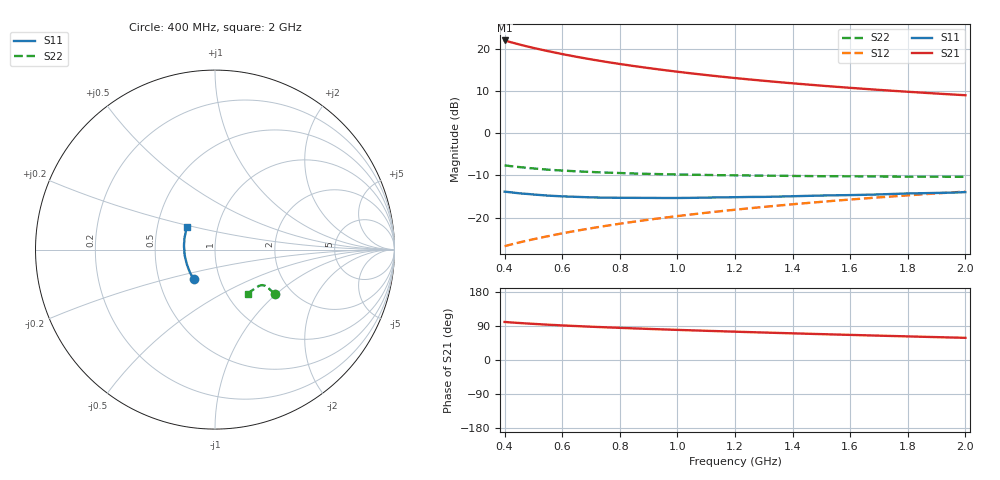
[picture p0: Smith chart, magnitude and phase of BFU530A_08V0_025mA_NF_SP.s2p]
! Filename:  P:\Prog\Test\Noise\ATS_data\Testdata_Net\06 Compressed Noise after Statistics\BFU530A_APG2013_33_A05_08p0V_025mA_NF_CM01_D.sf
! Date/Time: Tue 16/Apr/2013 15:10:58
! BFU530A_APG2013_33_A05_08p0V_1to25mA_NF_CM01_Bias8_R.sf
! Noise Parameter Data File
! BFU530A_APG2013_33_A05_08p0V_1to25mA_NF_CM01
! Date/time: Fri Apr 12 16:45:05 2013
! VAR V_out= 8.001000
! VAR I_out= 25.000000
! VAR V_in= 0.812800
! VAR I_in= 0.260050
! Device data file deembeded for feedlines and parallel
! Original file: \06 Compressed Noise after Statistics\BFU530A_APG2013_33_A05_08p0V_025mA_NF_CM01_R.sf
! Feed-files: PR017V01_150413_Feed1.s2p, PR017V01_150413_Feed2.s2p
! Parallel-file: PR017V01_150413_Par.s2p
# MHz S MA R 50
!  Freq-MHz  S11-mag  S11-arg  S21-mag  S21-arg  S12-mag  S12-arg  S22-mag  S22-arg
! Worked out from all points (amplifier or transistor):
!   37 points, 400 MHz to 2 GHz, reference 50 ohm
!   highest |S21| = 22.0 dB at 400 MHz (marker M1)
!   |S21| within 3 dB of that: start of sweep to 584 MHz
!   unconditionally stable (mu >= 1): 947.2 MHz to 1.909 GHz
!   at 500 MHz: K = 0.94, MSG = 22.7 dB, |S12| = -25.1 dB
!   at 1.1 GHz: K = 1.00, MAG = 15.9 dB, |S12| = -18.8 dB
!   at 2 GHz: K = 1.00, MSG = 11.4 dB, |S12| = -13.8 dB
!   lowest NFmin = 1.18 dB at 420 MHz
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400  0.203 -125.3  12.55 100.4  0.04593 73.0  0.4161 -36.6
420  0.1999 -128.1  12.01 99.2  0.04785 73.1  0.4078 -36.5
440  0.1962 -131.0  11.51 98.2  0.04976 73.2  0.4007 -36.4
480  0.1908 -135.7  10.63 96.2  0.05361 73.5  0.3881 -36.2
500  0.188 -138.2  10.24 95.4  0.05554 73.6  0.3829 -36.1
550  0.1824 -144.0  9.391 93.2  0.06028 73.9  0.3699 -35.8
600  0.1787 -148.8  8.655 91.3  0.06515 74.0  0.3612 -35.7
650  0.1762 -153.4  8.032 89.5  0.07003 74.1  0.3537 -35.8
700  0.1739 -157.6  7.492 87.8  0.07487 74.2  0.3476 -35.8
750  0.1723 -161.6  7.019 86.3  0.0798 74.2  0.3419 -35.9
800  0.1719 -165.2  6.607 84.8  0.0847 74.1  0.3378 -36.2
850  0.1716 -169.0  6.239 83.4  0.08955 74.0  0.3332 -36.5
900  0.1714 -172.4  5.91 82.0  0.09451 73.9  0.3297 -36.9
950  0.1709 -175.4  5.616 80.7  0.09939 73.8  0.3272 -37.3
1050  0.1716 178.8  5.106 78.2  0.1093 73.4  0.3223 -38.2
1100  0.1728 176.1  4.888 77.0  0.1142 73.2  0.3206 -38.8
1200  0.1746 171.1  4.503 74.7  0.1241 72.7  0.317 -40.0
1350  0.1776 164.2  4.033 71.4  0.139 71.8  0.3135 -42.1
1500  0.1828 157.9  3.658 68.3  0.1539 70.9  0.3097 -44.4
1650  0.1865 152.4  3.351 65.2  0.1689 69.8  0.308 -47.0
1750  0.1909 148.9  3.176 63.3  0.1787 69.0  0.3064 -48.7
2000  0.2005 141.4  2.817 58.5  0.2035 67.1  0.3046 -53.5
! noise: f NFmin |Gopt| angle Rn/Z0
400  1.222  0.2492  -167.4  0.0968
460  1.201  0.2855  -164.4  0.0809
600  1.248  0.2722  -157.5  0.1023
800  1.235  0.2971  -156.1  0.0891
1000  1.26  0.3092  -151.6  0.0911
1200  1.294  0.3173  -143.2  0.1039
1400  1.317  0.3286  -139.8  0.108
1600  1.345  0.3437  -134.4  0.1136
1800  1.328  0.3555  -132.3  0.124
2000  1.362  0.3666  -122.5  0.142
